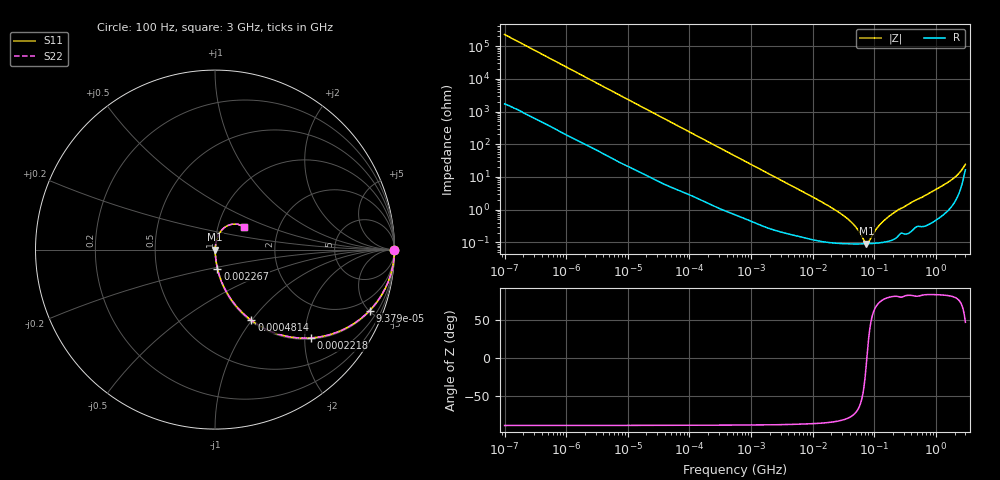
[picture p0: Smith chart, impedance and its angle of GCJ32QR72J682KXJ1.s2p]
!Murata Part Number: GCJ32QR72J682KXJ1
!These Parameters are Measured in Series Mode Connection
!Data Generated on Mar 13, 2026
!  o--ll--o
!Port1  Port2
!  o------o
!Operation Temp=25[degC], DC Bias Voltage=0[V]
!Freq. Start=100[Hz] Stop=3[GHz] 401[Steps]
# Hz S RI R 50
!Freq.(Hz) S11(Real) S11(Imag) S21(Real) S21(Imag) S12(Real) S12(Imag) S22(Real) S22(Imag)
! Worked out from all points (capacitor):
!   401 points, 100 Hz to 3 GHz, reference 50 ohm
!   read as one part in series: C = 6.98 nF near 109 Hz
!   lowest |Z| = 91.6 mohm at 74.05 MHz (marker M1)
!   series resonance near 75.64 MHz, so ESL is about 630 pH
!   S11 on the Smith chart (normalised r, x): 100 Hz: open; 93.79 kHz: 1.06, -5.05; 221.8 kHz: 1.03, -2.15; 481.4 kHz: 1.02, -1.00; 2.267 MHz: 1.00, -0.21; 3 GHz: 1.33, +0.35
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100  1 -0.000439  3.5e-06 0.000439  3.5e-06 0.000439  1 -0.000439
1788  0.9999 -0.00772  0.000126 0.00772  0.000126 0.00772  0.9999 -0.00772
10443  0.9976 -0.0446  0.00239 0.0446  0.00239 0.0446  0.9976 -0.0446
31977  0.9806 -0.1331  0.0194 0.1331  0.0194 0.1331  0.9806 -0.1331
93790  0.8615 -0.3395  0.1385 0.3395  0.1385 0.3395  0.8615 -0.3395
221826  0.5357 -0.4922  0.4643 0.4922  0.4643 0.4922  0.5357 -0.4922
481374  0.2027 -0.3943  0.7973 0.3943  0.7973 0.3943  0.2027 -0.3943
547723  0.1653 -0.3635  0.8347 0.3635  0.8347 0.3635  0.1653 -0.3635
1000599  0.0588 -0.2263  0.9412 0.2263  0.9412 0.2263  0.0588 -0.2263
2266852  0.0137 -0.1056  0.9863 0.1056  0.9863 0.1056  0.0137 -0.1056
9794414  0.00182 -0.0248  0.9982 0.0248  0.9982 0.0248  0.00182 -0.0248
2.21892e7  0.00105 -0.0102  0.9989 0.0102  0.9989 0.0102  0.00105 -0.0102
3.71925e7  0.000927 -0.00508  0.9991 0.00508  0.9991 0.00508  0.000927 -0.00508
5.026954e7  0.000902 -0.00277  0.9991 0.00277  0.9991 0.00277  0.000902 -0.00277
7.405258e7  0.000905 -0.000138  0.9991 0.000138  0.9991 0.000138  0.000905 -0.000138
8.070971e7  0.000911 0.00043  0.9991 -0.00043  0.9991 -0.00043  0.000911 0.00043
1.188943e8  0.000972 0.00309  0.999 -0.00309  0.999 -0.00309  0.000972 0.00309
1.751444e8  0.00114 0.00626  0.9989 -0.00626  0.9989 -0.00626  0.00114 0.00626
2.471375e8  0.00171 0.00989  0.9983 -0.00989  0.9983 -0.00989  0.00171 0.00989
1.573002e9  0.0139 0.067  0.9861 -0.067  0.9861 -0.067  0.0139 0.067
2.317205e9  0.0413 0.1127  0.9587 -0.1127  0.9587 -0.1127  0.0413 0.1127
3e9  0.1617 0.1274  0.8383 -0.1274  0.8383 -0.1274  0.1617 0.1274
